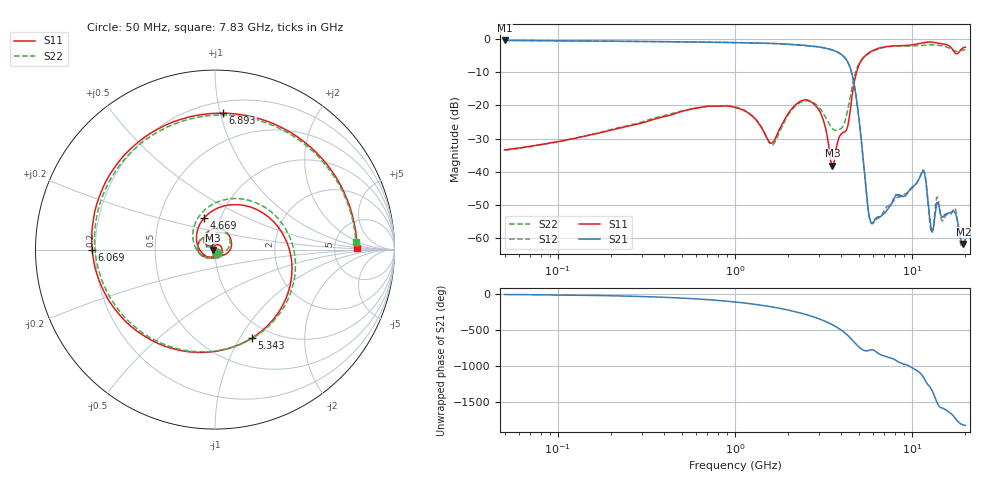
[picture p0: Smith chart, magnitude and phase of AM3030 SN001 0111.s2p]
# Hz S DB R 50
!freq MagS11 AngS11 MagS21 AngS21 MagS12 AngS12 MagS22 AngS22
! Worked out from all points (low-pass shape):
!   1601 points, 50 MHz to 20.05 GHz, reference 50 ohm
!   highest |S21| = -0.36 dB at 50 MHz (marker M1); lowest = -61.9 dB at 19.53 GHz (marker M2)
!   |S21| within 3 dB of the highest: start of sweep to 3.606 GHz
!   lowest |S11| = -38.2 dB at 3.552 GHz (marker M3), VSWR 1.02, Z = 48.8 - j0.148 ohm
!   |S11| at or under -10 dB: start of sweep to 4.863 GHz
!   |S22| runs from -33.4 to -1.7 dB; largest |S21 - S12| = 0.013
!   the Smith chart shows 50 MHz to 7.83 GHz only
!   S11 on the Smith chart (normalised r, x): 50 MHz: 1.02, -0.04; 4.669 GHz: 0.84, +0.31; 5.343 GHz: 0.82, -1.13; 6.069 GHz: 0.19, -0.00; 6.893 GHz: 0.28, +1.02; 7.83 GHz: 8.57, +0.31
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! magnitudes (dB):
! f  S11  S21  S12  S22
! 50 MHz  -33.4  -0.4  -0.4  -33.3
! 135.9 MHz  -29.5  -0.5  -0.5  -29.4
! 369.6 MHz  -23.8  -0.7  -0.7  -23.5
! 1.005 GHz  -20.6  -1.0  -1.0  -20.4
! 1.623 GHz  -31.3  -1.3  -1.3  -31.9
! 2.722 GHz  -19.1  -2.1  -2.1  -18.9
! 3.139 GHz  -24.0  -2.5  -2.5  -22.2
! 3.552 GHz  -38.2  -3.2  -3.3  -27.0
! 4.111 GHz  -28.1  -5.2  -5.2  -25.9
! 4.669 GHz  -14.6  -12.3  -12.3  -12.5
! 5.343 GHz  -5.5  -38.0  -38.0  -5.5
! 5.716 GHz  -4.1  -53.0  -53.1  -4.3
! 6.069 GHz  -3.3  -55.2  -55.5  -3.5
! 6.893 GHz  -2.4  -52.9  -52.2  -2.5
! 7.402 GHz  -2.1  -50.9  -50.3  -2.2
! 7.83 GHz  -2.0  -48.5  -49.1  -2.1
! 11.56 GHz  -1.1  -39.7  -39.5  -1.8
! 12.89 GHz  -0.8  -57.6  -58.4  -1.7
! 13.94 GHz  -1.2  -49.3  -47.8  -1.8
! 17.45 GHz  -4.0  -52.3  -51.1  -3.5
! 19.53 GHz  -2.5  -61.9  -61.7  -3.2
! 20.05 GHz  -2.4  -60.6  -60.0  -3.2
